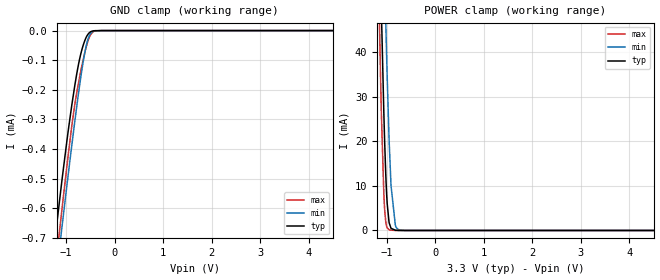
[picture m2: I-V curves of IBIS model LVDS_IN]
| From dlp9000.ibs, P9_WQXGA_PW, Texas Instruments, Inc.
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|   Model
[Model]   LVDS_IN
Model_type   Input
Vinl = 0.7
Vinh = 1.7
|   typ   min   max
C_comp   0.650pF   0.629pF   0.687pF
[Voltage Range]   3.3   3   3.6
[Temperature Range]   25   125   -40
[Power Clamp Reference]   3.3   3   3.6
[GND Clamp Reference]   -0   -0   -0
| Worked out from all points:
|   GND clamp passes 1 mA (typ) near -1.43 V on its own axis
|   POWER clamp passes 1 mA (typ) near -0.93 V on its own axis
[GND Clamp]
|   Voltage   I(typ)   I(min)   I(max)
-3.3V     -3.914mA   -3.944mA   -4.457mA
-1.231V   -705.2uA   -865.1uA   -814uA
-1.201V   -662.8uA   -822.9uA   -769.7uA
-1.092V   -511.2uA   -669.7uA   -609.4uA
-884.4mV  -250.7uA   -386.1uA   -320.8uA
-755.7mV  -121.4uA   -222.3uA   -184.5uA
-686.4mV  -70.18uA   -142.5uA   -126uA
-607.2mV  -29.7uA    -66.19uA   -67.54uA
-547.8mV  -11.58uA   -27.3uA    -33.22uA
-488.4mV  -3.319uA   -8.042uA   -11.51uA
-270.6mV  -1.983nA   -24.55nA   -5.471nA
6.59V     0A         0A         0A
[POWER Clamp]
|   Voltage   I(typ)   I(min)   I(max)
-3.3V     1.449A     1.486A     1.431A
-1.211V   102.3mA    146.5mA    77.15mA
-1.122V   53.88mA    96.62mA    30.32mA
-1.112V   48.94mA    91.32mA    25.86mA
-1.063V   26.5mA     65.82mA    8.302mA
-1.023V   12.75mA    47.09mA    1.982mA
-993.3mV  6.028mA    34.46mA    600.9uA
-953.7mV  1.753mA    20.26mA    167.8uA
-914.1mV  483.2uA    10.04mA    72.52uA
-825mV    57.01uA    1.168mA    9.199uA
-735.9mV  7.655uA    128.3uA    2.121uA
6.59V     0A         0A         0A
